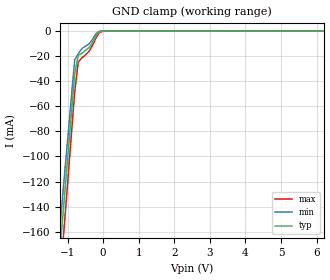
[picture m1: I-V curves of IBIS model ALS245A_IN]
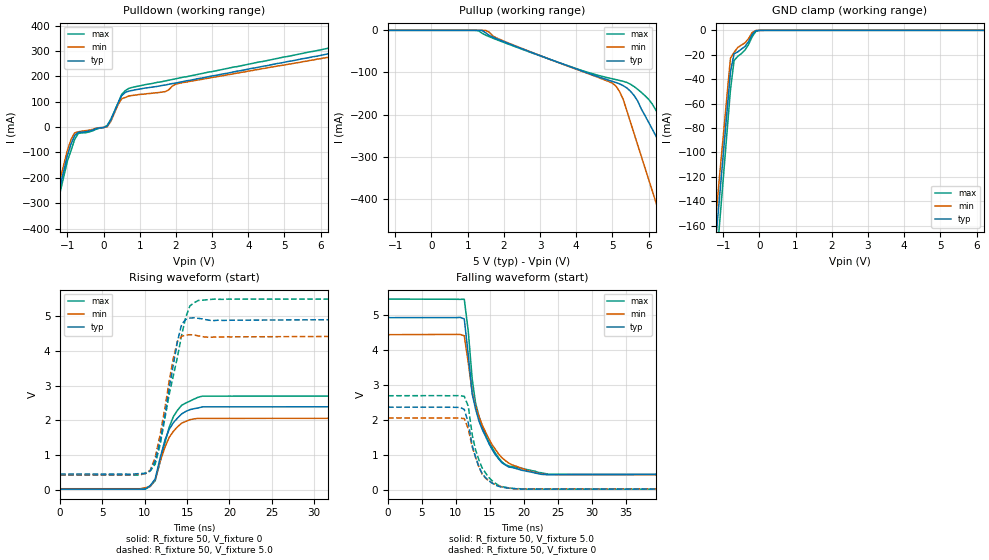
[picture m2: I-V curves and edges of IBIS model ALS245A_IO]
| TEXAS INSTRUMENTS INCORPORATED
| Standard Linear and Logic Group
| IBIS Model of SN74ALS245A
| OCTAL BUS TRANSCEIVERS WITH 3-STATE OUTPUTS
| SOIC 20-pin (DW), SOP 20-pin (NS), SSOP 20-pin (DB), P-DIP 20-pin (N) Package
[IBIS Ver]   3.2
[Comment Char]  |_char
[File Name]   sn74als245a.ibs
[File Rev]   4.1
[Date]   Sept.23, 2004
[Source]   Data created from Lab data at TI-SLL.
[Notes]   The following is an IBIS list for the ALS245A.
   Please contact sllibis@ti.com with questions and
   comments concerning SLL IBIS models.
   - FILE REV HISTORY
   - 4.1 Re-Release IBIS file on 09/27/04
   - Power clamp data deleted as there is no power-clamp diode.
   - Pullup and power clamp data modified to remove error
   when parsing with IBISCHK 3.2
   - Rise time and fall time data modified to remove error
   when parsing with IBISCHK 3.2
[Disclaimer] Property of Texas Instruments Incorporated.  Unauthorized
   reproduction and/or distribution is strictly prohibited.
   This product is protected under copyright law.
   Created 2000, (C) Copyright 2000, Texas Instruments Inc.,
   All Rights Reserved.
   UNLESS THERE IS A SIGNED, WRITTEN AGREEMENT TO THE
   CONTRARY, TEXAS INSTRUMENTS () IS PROVIDING THE IBIS
   MODELS  AND WITHOUT ANY WARRANTY, EXPRESSED OR
   IMPLIED.  TI assumes no liability for:
   1) the accuracy of the IBIS models provided to your
   company;
   2) the proper functioning of these IBIS Models in your
   design or for any resulting applications; or
   3) infringement of patents, copyrights or intellectual
   property rights resulting from your use of these IBIS
   models.
   TI provides IBIS Models as a service to our customers.
   You and your company shall not distribute, sell or give
   these models to anyone else without prior written
   permission from TI.
   TI reserves the right to make changes to our products or
   to discontinue any semiconductor product or service
   without notice, and advises our customers to obtain the
   latest version of relevant information to verify, before
   placing orders, that the information being relied on is
   current.
   Please be aware that your receipt and use of the IBIS
   information provided shall serve as acceptance of these
   terms and conditions.  If you do not accept these terms,
   you should return or destroy the IBIS models and any
   other accompanying information immediately.
|   Component ALS245A_DW
[Component]   ALS245A_DW
[Manufacturer]  Texas Instruments, Inc.
[Package]
|   typ   min   max
R_pkg   0.038   0.033   0.045
L_pkg   5.012nH   4.110nH   6.349nH
C_pkg   0.717pF   0.530pF   0.868pF
[Pin]   signal_name   model_name   R_pin   L_pin   C_pin
1   DIR   ALS245A_IN   0.042   6.336nH   0.865pF
2   A1   ALS245A_IO   0.043   5.542nH   0.867pF
3   A2   ALS245A_IO   0.034   4.714nH   0.732pF
4   A3   ALS245A_IO   0.034   4.377nH   0.591pF
5   A4   ALS245A_IO   0.036   4.130nH   0.533pF
6   A5   ALS245A_IO   0.035   4.111nH   0.530pF
7   A6   ALS245A_IO   0.034   4.284nH   0.583pF
8   A7   ALS245A_IO   0.034   4.634nH   0.726pF
9   A8   ALS245A_IO   0.040   5.518nH   0.865pF
10   GND   GND   0.043   6.349nH   0.866pF
11   B8   ALS245A_IO   0.041   6.281nH   0.861pF
12   B7   ALS245A_IO   0.045   5.561nH   0.868pF
13   B6   ALS245A_IO   0.033   4.778nH   0.742pF
14   B5   ALS245A_IO   0.035   4.414nH   0.596pF
15   B4   ALS245A_IO   0.035   4.110nH   0.533pF
16   B3   ALS245A_IO   0.036   4.130nH   0.533pF
17   B2   ALS245A_IO   0.034   4.377nH   0.591pF
18   B1   ALS245A_IO   0.034   4.714nH   0.731pF
19   OE_NOT   ALS245A_IN   0.043   5.569nH   0.868pF
20   VCC   POWER   0.042   6.308nH   0.864pF
|   Component ALS245A_NS
[Component]   ALS245A_NS
[Manufacturer]  Texas Instruments, Inc.
[Package]
|   typ   min   max
R_pkg   0.044   0.029   0.058
L_pkg   3.666nH   2.317nH   5.115nH
C_pkg   0.548pF   0.316pF   0.725pF
[Pin]   signal_name   model_name   R_pin   L_pin   C_pin
1   DIR   ALS245A_IN   0.058   5.115nH   0.725pF
2   A1   ALS245A_IO   0.053   4.591nH   0.724pF
3   A2   ALS245A_IO   0.049   3.754nH   0.572pF
4   A3   ALS245A_IO   0.029   2.549nH   0.388pF
5   A4   ALS245A_IO   0.031   2.317nH   0.316pF
6   A5   ALS245A_IO   0.031   2.317nH   0.316pF
7   A6   ALS245A_IO   0.029   2.556nH   0.399pF
8   A7   ALS245A_IO   0.049   3.754nH   0.579pF
9   A8   ALS245A_IO   0.053   4.591nH   0.724pF
10   GND   GND   0.058   5.115nH   0.725pF
11   B8   ALS245A_IO   0.058   5.115nH   0.725pF
12   B7   ALS245A_IO   0.053   4.591nH   0.724pF
13   B6   ALS245A_IO   0.049   3.754nH   0.579pF
14   B5   ALS245A_IO   0.029   2.557nH   0.399pF
15   B4   ALS245A_IO   0.031   2.317nH   0.316pF
16   B3   ALS245A_IO   0.031   2.317nH   0.316pF
17   B2   ALS245A_IO   0.029   2.557nH   0.399pF
18   B1   ALS245A_IO   0.049   3.754nH   0.579pF
19   OE_NOT   ALS245A_IN   0.053   4.591nH   0.724pF
20   VCC   POWER   0.058   5.115nH   0.725pF
|   Component ALS245A_DB
[Component]   ALS245A_DB
[Manufacturer]  Texas Instruments, Inc.
[Package]
|   typ   min   max
R_pkg   0.040   0.035   0.051
L_pkg   3.495nH   3.035nH   4.314nH
C_pkg   0.420pF   0.346pF   0.502pF
[Pin]   signal_name   model_name   R_pin   L_pin   C_pin
1   DIR   ALS245A_IN   0.049   4.310nH   0.502pF
2   A1   ALS245A_IO   0.048   3.903nH   0.487pF
3   A2   ALS245A_IO   0.035   3.189nH   0.396pF
4   A3   ALS245A_IO   0.035   3.036nH   0.347pF
5   A4   ALS245A_IO   0.035   3.035nH   0.367pF
6   A5   ALS245A_IO   0.035   3.035nH   0.367pF
7   A6   ALS245A_IO   0.035   3.036nH   0.347pF
8   A7   ALS245A_IO   0.035   3.189nH   0.397pF
9   A8   ALS245A_IO   0.047   3.899nH   0.488pF
10   GND   GND   0.051   4.314nH   0.500pF
11   B8   ALS245A_IO   0.051   4.314nH   0.500pF
12   B7   ALS245A_IO   0.047   3.899nH   0.488pF
13   B6   ALS245A_IO   0.035   3.189nH   0.397pF
14   B5   ALS245A_IO   0.035   3.036nH   0.346pF
15   B4   ALS245A_IO   0.035   3.035nH   0.367pF
16   B3   ALS245A_IO   0.035   3.035nH   0.367pF
17   B2   ALS245A_IO   0.035   3.036nH   0.346pF
18   B1   ALS245A_IO   0.035   3.189nH   0.397pF
19   OE_NOT   ALS245A_IN   0.047   3.899nH   0.488pF
20   VCC   POWER   0.051   4.314nH   0.502pF
|   Component ALS245A_N
[Component]   ALS245A_N
[Manufacturer]  Texas Instruments, Inc.
[Package]
|   Mean.   Min.   Max.
R_pkg   0.043   0.038   0.05
L_pkg   7.384nH   4.68nH   10.321nH
C_pkg   0.51pF   0.231pF   0.821pF
[Pin]   signal_name   model_name   R_pin   L_pin   C_pin
1   DIR   ALS245A_IN   0.042   9.427nH   0.81pF
2   A1   ALS245A_IO   0.046   8.544nH   0.456pF
3   A2   ALS245A_IO   0.048   7.163nH   0.435pF
4   A3   ALS245A_IO   0.04   4.825nH   0.261pF
5   A4   ALS245A_IO   0.04   5.284nH   0.648pF
6   A5   ALS245A_IO   0.04   4.686nH   0.232pF
7   A6   ALS245A_IO   0.04   6.359nH   0.489pF
8   A7   ALS245A_IO   0.038   7.982nH   0.475pF
9   A8   ALS245A_IO   0.043   9.403nH   0.475pF
10   GND   GND   0.05   10.321nH  0.805pF
11   B8   ALS245A_IO   0.05   10.281nH  0.81pF
12   B7   ALS245A_IO   0.043   9.383nH   0.477pF
13   B6   ALS245A_IO   0.038   7.978nH   0.476pF
14   B5   ALS245A_IO   0.04   6.302nH   0.492pF
15   B4   ALS245A_IO   0.04   4.68nH   0.231pF
16   B3   ALS245A_IO   0.04   5.284nH   0.648pF
17   B2   ALS245A_IO   0.04   4.822nH   0.261pF
18   B1   ALS245A_IO   0.047   7.118nH   0.439pF
19   OE_NOT   ALS245A_IN   0.046   8.492nH   0.461pF
20   VCC   POWER   0.043   9.348nH   0.821pF
| Models and submodels in the file (2): ALS245A_IN (Input), ALS245A_IO (I/O)
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|   Model ALS245A_IN
[Model]   ALS245A_IN
Model_type  Input
Polarity   Inverting
Vinl = 0.8
Vinh = 2.0
| variable   typ   min   max
C_comp   1.30pf   0.98pf   1.62pf
[Temperature Range]   25   0   70
[Voltage Range]   5.0   4.5   5.5
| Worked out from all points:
|   GND clamp passes 1 mA (typ) near -0.12 V on its own axis
[GND Clamp]
|   Voltage   I(typ)   I(min)   I(max)
-5V       -1.46A     -1.38A     -1.58A
-1.3V     -204mA     -184mA     -231mA
-1.2V     -170mA     -152mA     -194mA
-1.1V     -136mA     -119mA     -158mA
-800mV    -34.1mA    -22.8mA    -48.8mA
-700mV    -19.2mA    -18.1mA    -24.7mA
-600mV    -17.7mA    -14.1mA    -21.4mA
-400mV    -13.3mA    -10.3mA    -16.2mA
-300mV    -9.23mA    -6.8mA     -11.6mA
-200mV    -3.42mA    -1.87mA    -5.23mA
-100mV    -337uA     -107uA     -887uA
10V       4.9nA      356pA      66.1nA
|   Model ALS245A_IO
[Model]   ALS245A_IO
Model_type  I/O
Polarity   Non-Inverting
Enable   Active-Low
Vinl = 0.8
Vinh = 2.0
Vmeas = 2.5v
Cref = 15pf
| variable   typ   min   max
C_comp   6.0pf   4.5pf   7.5pf
[Temperature Range]   25   0   70
[Voltage Range]   5.0   4.5   5.5
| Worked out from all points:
|   slope of the pulldown table from 0 to 0.75 V, typ, clamps not added: 5.16 ohm
|   GND clamp passes 1 mA (typ) near -0.12 V on its own axis
|   rising waveform, R_fixture 50, V_fixture 0: 20-80 % time 1.94ns typ, 1.9ns min, 1.99ns max; typ from 0.021 V to 2.4 V
|   falling waveform, R_fixture 50, V_fixture 5.0: 20-80 % time 3.08ns typ, 3.72ns min, 2.88ns max; typ from 4.93 V to 0.457 V
|   rising waveform, R_fixture 50, V_fixture 5.0: 20-80 % time 1.94ns typ, 1.76ns min, 2.46ns max; typ from 0.457 V to 4.93 V
|   falling waveform, R_fixture 50, V_fixture 0: 20-80 % time 1.96ns typ, 2ns min, 2.13ns max; typ from 2.37 V to 0.024 V
[Pulldown]
|   Voltage   I(typ)   I(min)   I(max)
-5V       -2.5A      -2.37A     -2.57A
-1.6V     -471mA     -433mA     -500mA
-1.5V     -411mA     -376mA     -439mA
-1.4V     -351mA     -319mA     -378mA
-1V       -112mA     -91.6mA    -134mA
-800mV    -33.3mA    -22.6mA    -48.6mA
-700mV    -20.3mA    -18.6mA    -24.8mA
100mV     4.23mA     1.64mA     6.86mA
500mV     124mA      112mA      129mA
700mV     142mA      123mA      153mA
8.8V      359mA      340mA      385mA
10V       392mA      369mA      420mA
[Pullup]
|   Voltage   I(typ)   I(min)   I(max)
-5V       83.86nA    4.695nA    1.221uA
1.2V      -306.6nA   3.724nA    -58.91uA
1.5V      -5.829mA   -211uA     -11.57mA
5.1V      -123.9mA   -132.5mA   -117mA
5.3V      -131.4mA   -164.2mA   -121mA
5.6V      -154.7mA   -245.3mA   -133.5mA
6V        -218.2mA   -353.5mA   -163.7mA
6.4V      -282.6mA   -461.7mA   -218.5mA
7V        -379.2mA   -623.9mA   -305.9mA
7.6V      -475.8mA   -786.1mA   -393.4mA
8.2V      -572.4mA   -948.4mA   -480.9mA
10V       -862.2mA   -1.435A    -743.3mA
[GND Clamp]
|   Voltage   I(typ)   I(min)   I(max)
-5V       -1.46A     -1.38A     -1.58A
-1.3V     -204mA     -184mA     -231mA
-1.2V     -170mA     -152mA     -194mA
-1.1V     -136mA     -119mA     -158mA
-800mV    -34.1mA    -22.8mA    -48.8mA
-700mV    -19.2mA    -18.1mA    -24.7mA
-600mV    -17.7mA    -14.1mA    -21.4mA
-400mV    -13.3mA    -10.3mA    -16.2mA
-300mV    -9.23mA    -6.8mA     -11.6mA
-200mV    -3.42mA    -1.87mA    -5.23mA
-100mV    -337uA     -107uA     -887uA
10V       4.9nA      356pA      66.1nA
[Ramp]
| variable   typ   min   max
dV/dt_r  1.398E+00/1.968E-09  1.206E+00/1.946E-09  1.584E+00/1.914E-09
dV/dt_f  2.754E+00/3.153E-09  2.460E+00/3.805E-09  3.030E+00/2.874E-09
R_load = 50
[Rising Waveform]
R_fixture = 50
V_fixture = 0
V_fixture_min = 0
V_fixture_max = 0
C_fixture = 0pf
L_fixture = 0nH
|   Time   V(typ)   V(min)   V(max)
0s        21.06mV    32.34mV    20.06mV
10.06ns   26.16mV    62.48mV    21.75mV
10.64ns   122.1mV    98.27mV    100.4mV
11.23ns   314.3mV    291.4mV    265.2mV
12.4ns    1.448V     1.241V     1.375V
12.89ns   1.747V     1.515V     1.81V
13.38ns   1.937V     1.687V     2.112V
14.36ns   2.19V      1.924V     2.437V
16.8ns    2.392V     2.06V      2.701V
50ns      2.398V     2.063V     2.705V
[Falling Waveform]
R_fixture = 50
V_fixture = 5.0
V_fixture_min = 4.5
V_fixture_max = 5.5
C_fixture = 0pf
L_fixture = 0nH
|   Time   V(typ)   V(min)   V(max)
0s        4.928V     4.44V      5.459V
11.23ns   4.891V     4.41V      5.454V
11.82ns   3.857V     3.637V     4.534V
12.4ns    2.739V     2.795V     3.168V
12.89ns   2.318V     2.397V     2.491V
13.87ns   1.729V     1.856V     1.825V
14.84ns   1.332V     1.467V     1.384V
17.29ns   710.8mV    837mV      723.7mV
23.14ns   439.9mV    441.4mV    468.3mV
50ns      457.2mV    437.2mV    425.6mV
[Rising Waveform]
R_fixture = 50
V_fixture = 5.0
V_fixture_min = 4.5
V_fixture_max = 5.5
C_fixture = 0pf
L_fixture = 0nH
|   Time   V(typ)   V(min)   V(max)
0s        457.2mV    437.9mV    426.5mV
10.64ns   546mV      563.8mV    544.1mV
11.23ns   836.8mV    936.9mV    739.5mV
11.82ns   1.423V     1.594V     1.312V
13.38ns   3.618V     3.801V     3.297V
13.87ns   4.287V     4.284V     3.841V
14.36ns   4.778V     4.425V     4.466V
15.33ns   4.952V     4.472V     5.301V
16.31ns   4.944V     4.439V     5.458V
50ns      4.927V     4.44V      5.499V
[Falling Waveform]
R_fixture = 50
V_fixture = 0
V_fixture_min = 0
V_fixture_max = 0
C_fixture = 0pf
L_fixture = 0nH
|   Time   V(typ)   V(min)   V(max)
0s        2.366V     2.057V     2.693V
11.23ns   2.301V     2.04V      2.676V
11.82ns   1.923V     1.746V     2.395V
12.4ns    1.265V     1.23V      1.576V
12.89ns   937.8mV    932.5mV    1.147V
13.87ns   464.9mV    447.7mV    627.9mV
15.33ns   195.5mV    198.2mV    262.2mV
16.8ns    73.09mV    86.44mV    91.71mV
19.73ns   24.08mV    30mV       20.1mV
50ns      24mV       30.06mV    20.43mV
